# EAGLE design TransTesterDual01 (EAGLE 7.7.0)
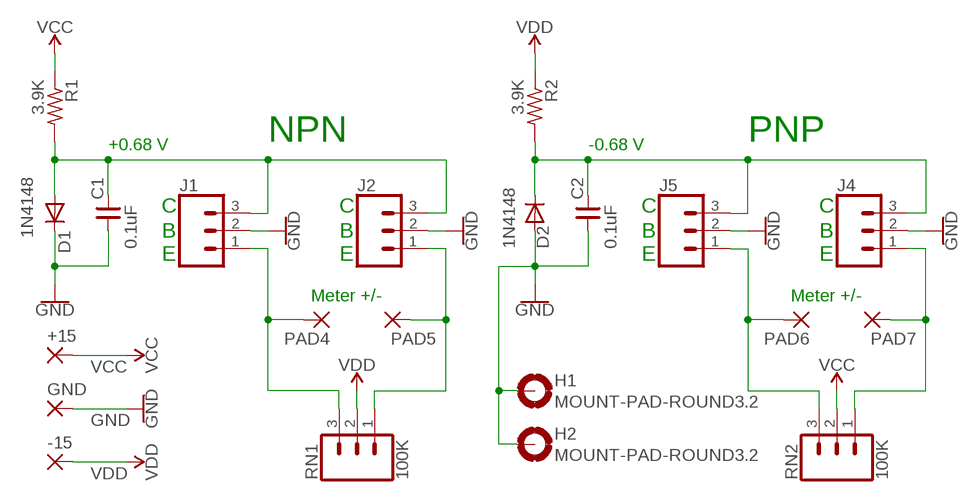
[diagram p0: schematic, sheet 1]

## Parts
+15  WIREPAD3,17/1,3  [3,17/1,3]
-15  WIREPAD3,17/1,3  [3,17/1,3]
C1  0.1uF  CNP-C025-050X025  [C025-050X025]
C2  0.1uF  CNP-C025-050X025  [C025-050X025]
D1  1N4148  1N4148DO35-7  [DO35-7]
D2  1N4148  1N4148DO35-7  [DO35-7]
GND  WIREPAD3,17/1,3  [3,17/1,3]
H1  MOUNT-PAD-ROUND3.2  [3,2-PAD]
H2  MOUNT-PAD-ROUND3.2  [3,2-PAD]
J1  CONN_031X03_NO_SILK  [1X03_NO_SILK]
J2  CONN_031X03_NO_SILK  [1X03_NO_SILK]
J4  CONN_031X03_NO_SILK  [1X03_NO_SILK]
J5  CONN_031X03_NO_SILK  [1X03_NO_SILK]
PAD4  WIREPAD3,17/1,3  [3,17/1,3]
PAD5  WIREPAD3,17/1,3  [3,17/1,3]
PAD6  WIREPAD3,17/1,3  [3,17/1,3]
PAD7  WIREPAD3,17/1,3  [3,17/1,3]
R1  3.9K  R-US_0207/7  [0207/7]
R2  3.9K  R-US_0207/7  [0207/7]
RN1  100K  CONN_031X03_NO_SILK  [1X03_NO_SILK]
RN2  100K  CONN_031X03_NO_SILK  [1X03_NO_SILK]

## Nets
GND: C1.1 C2.1 D1.C D2.A GND.1(P) H1.B3,2(MOUNT) H2.B3,2(MOUNT) J1.2 J2.2 J4.2 J5.2
N$1: C1.2 D1.A J1.3 J2.3 R1.2
N$3: J1.1 PAD4.1(P) RN1.3
N$4: J2.1 PAD5.1(P) RN1.1
N$6: C2.2 D2.C J4.3 J5.3 R2.2
N$8: J5.1 PAD6.1(P) RN2.3
N$9: J4.1 PAD7.1(P) RN2.1
VCC: +15.1(P) R1.1 RN2.2
VDD: -15.1(P) R2.1 RN1.2

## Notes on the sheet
- NPN | PNP
- +0.68 V | -0.68 V
- C | C | C | C
- B | B | B | B
- E | E | E | E
- Meter +/- | Meter +/-

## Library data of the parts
+15 -15 GND PAD4-PAD7 = wirepad:WIREPAD: Wire PAD connect wire on PCB
C1 C2 = cap-master:CNP-: NON-POLARIZED CAP
D1 D2 = diode:1N4148: DIODE
H1 H2 = holes:MOUNT-PAD-ROUND: MOUNTING PAD, round
J1 J2 J4 J5 RN1 RN2 = SparkFun-Connectors:CONN_03: Multi connection point. Often used as Generic Header-pin footprint for 0.1 inch spaced/style header connections On any of the 0.1 inch spaced packages, you can populate with these: Break Away Headers - Straight (PRT-00116) Break Away Male Headers - Right Angle (PRT-00553) Female Headers (PRT-00115)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
R1 R2 = resistor:R-US_: RESISTOR, American symbol

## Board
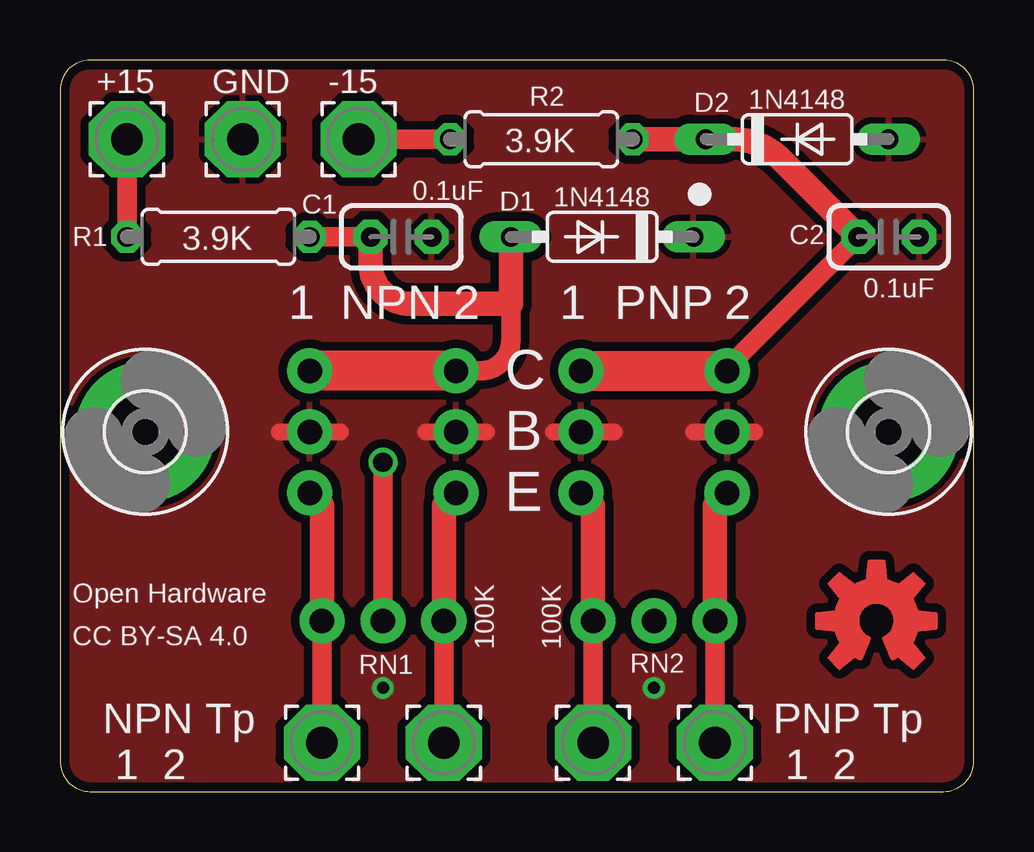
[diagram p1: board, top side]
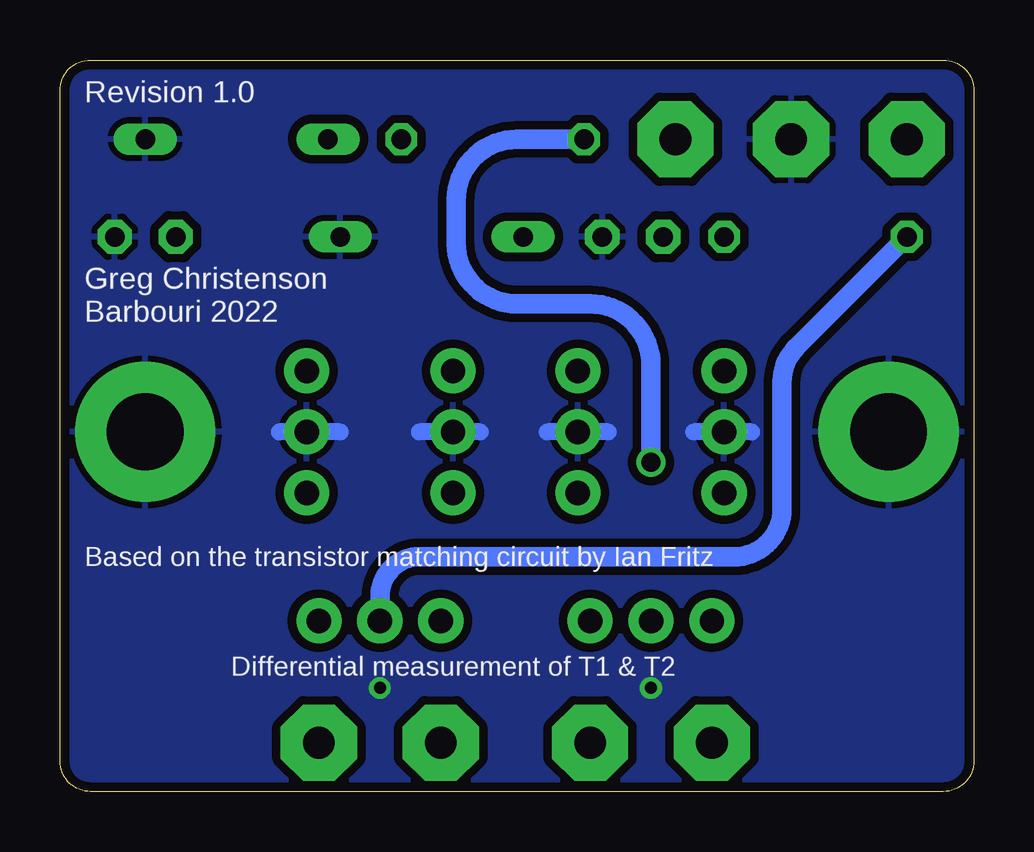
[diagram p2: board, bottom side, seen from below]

Size 38.1 x 30.48 mm. Coordinates in mm from the lower left corner, seen from the top.
Outline: 0,29.21 0,1.27 arc90 1.27,0 36.83,0 arc90 38.1,1.27 38.1,29.21 arc90 36.83,30.48 1.27,30.48 arc90 0,29.21
Copper layers (1*16): Top 0.035mm / dielectric 1.5mm / Bottom 0.035mm
Design rules "default *": minimum track width 10mil, minimum drill 9mil, track to track 14mil, track to pad 14mil, pad to pad 14mil, via to via 14mil, smd to smd 8mil, copper to edge 15mil, drill to drill 9mil, minimum pad ring 10mil, minimum via ring 8mil, stop-mask expansion 4mil, vias tented up to drill 20mil, thermal gap 10mil

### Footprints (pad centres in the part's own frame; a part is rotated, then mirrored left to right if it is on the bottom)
3,17/1,3 = drill 1.321 pad 3.175 octagon: 1 0,0
C025-050X025 = drill 0.813 pad 1.422 octagon: 1 -1.27,0; 2 1.27,0
DO35-7 = drill 0.813 long: A 3.81,0; C -3.81,0
3,2-PAD = drill 3.2 pad 5.842: B3,2 0,0
1X03_NO_SILK = drill 1.016 pad 1.88: 1 0,0; 2 2.54,0; 3 5.08,0
0207/7 = drill 0.813 octagon: 1 -3.81,0; 2 3.81,0

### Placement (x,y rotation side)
+15  2.79,27.18 0 top
-15  12.45,27.18 0 top
C1  14.22,23.11 180 top
C2  34.54,23.11 180 top
D1  22.61,23.11 180 top
D2  30.73,27.18 0 top
GND  7.62,27.18 0 top
H1  34.54,14.99 0 top
H2  3.56,14.99 0 top
J1  10.41,12.45 90 top
J2  16.51,12.45 90 top
J4  21.72,12.45 90 top
J5  27.81,12.45 90 top
PAD4  10.92,2.03 0 top
PAD5  16,2.03 0 top
PAD6  27.3,2.03 0 top
PAD7  22.23,2.03 0 top
R1  6.6,23.11 0 top
R2  20.07,27.18 0 top
RN1  16,7.11 180 top
RN2  22.23,7.11 0 top
U$1  [OSHW-LOGO-M_COPPER]  34.04,7.11 0 top

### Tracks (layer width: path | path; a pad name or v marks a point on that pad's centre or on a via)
GND  (via drill 0.5)
  Top 0.711: 15.24,14.99 17.78,14.99 | 9.14,14.99 11.68,14.99 | 20.57,14.99 23.11,14.99 | 26.42,14.99 28.96,14.99
  Bottom 0.711: 9.27,14.99 11.68,14.99 | 15.24,14.99 17.78,14.99 | 20.57,14.99 23.11,14.99 | 26.42,14.99 28.96,14.99
  other vias: 13.46,4.32 24.77,4.32
  pour Bottom: 0,0 38.1,0 38.1,30.48 0,30.48
  pour Top: 0,0 38.1,0 38.1,30.48 0,30.48
N$1
  Top 0.813: 18.8,20.32 18.8,18.8 arc-90 17.53,17.53 J2.3 | R1.2 C1.2
  Top 1.016: D1.A 18.8,20.32 14.61,20.32 arc-90 12.95,21.97 C1.2
  Top 1.676: J2.3 J1.3
N$3
  Top 0.813: PAD4.1 RN1.3
  Top 1.016: RN1.3 10.92,9.65 10.92,11.94 J1.1
N$4
  Top 0.406: 16,9.65 16,9.91
  Top 0.813: PAD5.1 RN1.1
  Top 1.016: RN1.1 16,9.91 16,11.94 J2.1
N$6
  Top 0.813: J5.3 27.94,17.78 C2.2
  Top 1.016: R2.2 D2.C 27.92,27.18 arc-45 29.94,26.45 C2.2
  Top 1.676: J4.3 J5.3
N$8
  Top 0.813: PAD6.1 RN2.3
  Top 1.016: RN2.3 27.3,11.94 J5.1
N$9
  Top 0.813: PAD7.1 RN2.1
  Top 1.016: RN2.1 22.23,11.94 J4.1
VCC
  Top 0.813: +15.1 R1.1
  Bottom 0.813: R1.1 7.42,18.49 arc-45 8,17.08 8,11.78 arc90 10,9.78 23.11,9.78 arc-90 24.77,8.13 RN2.2
VDD  (via drill 0.8)
  Top 0.813: -15.1 R2.1 | v13.46,13.72 RN1.2
  Bottom 0.813: v13.46,13.72 13.46,17.78 arc-90 16,20.32 19.05,20.32 arc90 21.59,22.86 21.59,24.64 arc90 19.05,27.18 R2.1

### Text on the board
tNames: 1 | NPN | 2 | 1 | PNP | 2 | C | B | E | Open Hardware | CC BY-SA 4.0 | NPN Tp / 1 2 | PNP Tp / 1 2
bNames: Revision 1.0 | Greg Christenson / Barbouri 2022 | Based on the transistor matching circuit by Ian Fritz | Differential measurement of T1 & T2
